// ================================================================================
// Automatically generated by   S5/S7 Converter,  Version K2.1.9.0-REL   12-04-2006 21:34
// ================================================================================
//
//                       Notes:
//                       ------
//
// BLOCKS:       The following block types exist in S7:
//OB: as in STEP 5;
//FB: function block (for example, closed-loop controller), is called using different instance data blocks;
//FC: function, similar to STEP 5 FBs.
//The block types PB, FX, DX and SB no longer exist.
//
//OBS:   OBs cannot be called from the user program in S7.
//        Special function OBs can be replaced by new instructions or by SFCs
//             in the same way as special instructions such as G DB.
//
// ADDRESSING: In S7, all memory areas (I, Q, M, D, etc.) can be addressed
//             as bytes. This means L DW 2 in S5 becomes L DBW 4 in S7.
//
// NO. OF ACCUS: All S7 CPUs have either 2 or 4 accumulators just as the S5 CPUs.
//               If an S5 program from an S5 CPU with 2 accumulators (S5-115U) is converted for an S7 CPU
//               with 4 accumulators, an ENT instruction must be added in front
//               of every math operation (+,-,*,/) in case the contents of accumulator 2
//               are to be used again afterwards.
//
// ACCU WIDTH: The accumulators of all S7 CPUs are 32 bits wide.
//             With fixed-point math operations in S7
//              - the high word in accumulator 1 remains unchanged following overflow/underflow
//                (S5-135U: sign);
//              - no implicit conversion to 32-bit format is performed (S5-155U).
//
// OS BIT:     With the following operations in S7, the OS bit
//             (stored overflow) remains unchanged (in S5 it was reset):
//             T,  >F, <F, ><F, !=F, >=F, <=F,  >D, <D, ><D, !=D, >=D, <=D,
//             >G, <G, ><G, !=G, >=G, <=G,
//             SLW, SRW, SLD, SSW, SSD, RLD, RRD
//
// OV BIT:      The following conversion operations leave the accumulator 1 unchanged
//              following an overflow (in S5: value of fixed-point number).
//              An overflow is displayed in the OS and OV bit (S5: only OS).
//              DUF, DUD, GFD
//
// LIR, TIR:    In S7 there are no instructions for absolute addressing. They are
//              partly replaced by new instructions (for example, access to data words greater than 255),
//              and partly by system functions (SFCs). The same applies to
//              data block start, data block length, and base register.
//
// DATA AREAS RS, RT, RI, RJ, Q:
//              When these data areas are used, the conversion requires manual assistance.
//              Possible solutions:
//                 - use the extended bit memory area
//                 - define longer data blocks
//                 - use S7 system functions (SFCs)
//
// STOP INSTRUCTIONS: In S7 there is only one stop instruction which can be executed by means of an
//               SFC call. It corresponds to the STS operation in S5.
//
// Refer to the manual or the on-line help for further information.


ORGANIZATION_BLOCK OB 1
VAR_TEMP
  OB1_EV_CLASS : BYTE ; //Bits 0-3 = 1 (Coming event), Bits 4-7 = 1 (Event class 1)
  OB1_SCAN_1 : BYTE ;   //1 (Cold restart scan 1 of OB 1), 3 (Scan 2-n of OB 1)
  OB1_PRIORITY : BYTE ; //1 (Priority of 1 is lowest)
  OB1_OB_NUMBR : BYTE ; //1 (Organization block 1, OB1)
  OB1_RESERVED_1 : BYTE ;   //Reserved for system
  OB1_RESERVED_2 : BYTE ;   //Reserved for system
  OB1_PREV_CYCLE : INT ;    //Cycle time of previous OB1 scan (milliseconds)
  OB1_MIN_CYCLE : INT ; //Minimum cycle time of OB1 (milliseconds)
  OB1_MAX_CYCLE : INT ; //Maximum cycle time of OB1 (milliseconds)
  OB1_DATE_TIME : DATE_AND_TIME ;   //Date and time OB1 started
  END_VAR
  BEGIN
  NETWORK
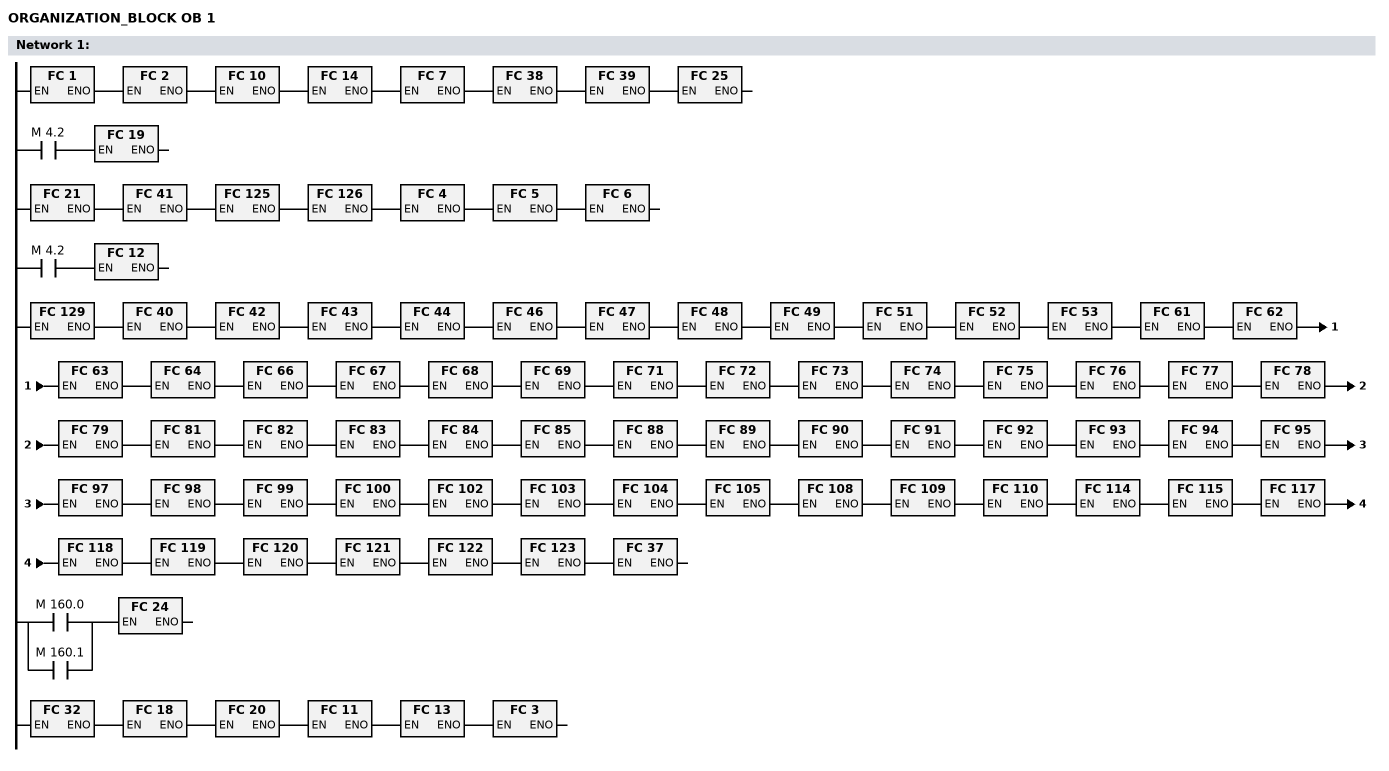
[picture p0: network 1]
       CALL FC 1;
       //;
       CALL FC 2;
       //;
       CALL FC 10;
       //;
       CALL FC 14;
       //;
       CALL FC 7;
       //;
       CALL FC 38;
       CALL FC 39;
       //;
       CALL FC 25;
       //;
       A   M 4.2;
       JCN   X000;
     CALL FC 19;
  X000: NOP 0;
       //;
       CALL FC 21;
       //;
       CALL FC 41;
       CALL FC 125;
       CALL FC 126;
       //;
       CALL FC 4;
       //;
       CALL FC 5;
       //;
       CALL FC 6;
       //;
       A   M 4.2;
       JCN   X001;
     CALL FC 12;
  X001: NOP 0;
       //;
       //;
       //;
       CALL FC 129;
       //;
       CALL FC 40;
       //;
       CALL FC 42;
       CALL FC 43;
       CALL FC 44;
       CALL FC 46;
       CALL FC 47;
       CALL FC 48;
       CALL FC 49;
       //;
       CALL FC 51;
       CALL FC 52;
       CALL FC 53;
       //;
       //;
       //;
       CALL FC 61;
       CALL FC 62;
       CALL FC 63;
       CALL FC 64;
       //;
       CALL FC 66;
       CALL FC 67;
       CALL FC 68;
       CALL FC 69;
       CALL FC 71;
       CALL FC 72;
       CALL FC 73;
       CALL FC 74;
       CALL FC 75;
       CALL FC 76;
       CALL FC 77;
       CALL FC 78;
       CALL FC 79;
       //;
       CALL FC 81;
       CALL FC 82;
       CALL FC 83;
       CALL FC 84;
       CALL FC 85;
       //;
       //;
       //;
       CALL FC 88;
       CALL FC 89;
       CALL FC 90;
       CALL FC 91;
       CALL FC 92;
       CALL FC 93;
       CALL FC 94;
       CALL FC 95;
       CALL FC 97;
       CALL FC 98;
       CALL FC 99;
       CALL FC 100;
       //;
       CALL FC 102;
       CALL FC 103;
       CALL FC 104;
       CALL FC 105;
       //;
       //;
       CALL FC 108;
       CALL FC 109;
       CALL FC 110;
       //;
       //;
       CALL FC 114;
       CALL FC 115;
       //;
       CALL FC 117;
       CALL FC 118;
       CALL FC 119;
       //;
       CALL FC 120;
       CALL FC 121;
       CALL FC 122;
       CALL FC 123;
       CALL FC 37;
       //;
       O   M 160.0;
       O   M 160.1;
       JCN   X002;
     CALL FC 24;
  X002: NOP 0;
       //;
       CALL FC 32;
       //;
       CALL FC 18;
       //;
       CALL FC 20;
       //;
       CALL FC 11;
       //;
       CALL FC 13;
       //;
       CALL FC 3;
       //;
  NETWORK


END_ORGANIZATION_BLOCK

ORGANIZATION_BLOCK OB 35
    // *** Warning in Line    5743:  Please check setting for time base (S7 Config.).
VAR_TEMP
  OB35_EV_CLASS : BYTE ;    //Bits 0-3 = 1 (Coming event), Bits 4-7 = 1 (Event class 1)
  OB35_STRT_INF : BYTE ;    //16#36 (OB 35 has started)
  OB35_PRIORITY : BYTE ;    //11 (Priority of 1 is lowest)
  OB35_OB_NUMBR : BYTE ;    //35 (Organization block 35, OB35)
  OB35_RESERVED_1 : BYTE ;  //Reserved for system
  OB35_RESERVED_2 : BYTE ;  //Reserved for system
  OB35_PHASE_OFFSET : WORD ;    //Phase offset (msec)
  OB35_RESERVED_3 : INT ;   //Reserved for system
  OB35_EXC_FREQ : INT ; //Frequency of execution (msec)
  OB35_DATE_TIME : DATE_AND_TIME ;  //Date and time OB35 started
  END_VAR
  BEGIN
  NETWORK
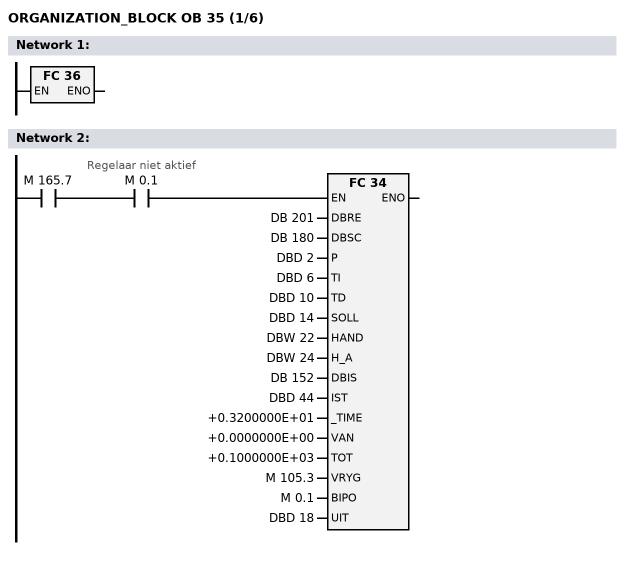
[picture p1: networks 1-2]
       CALL FC 36;
  NETWORK
       A   M 165.7;
       A   M 0.1;                // Regelaar niet aktief
       JCN   X000;

//  NAME: REGELAAR
//  VAR_INPUT
//    DBRE      :block_db;  // DBRE
//    DBSC      :block_db;  // DBSC
//    P         :dword;     // P
//    TI        :dword;     // TI
//    TD        :dword;     // TD
//    SOLL      :dword;     // SOLL
//    HAND      :word;      // HAND
//    H_A       :word;      // H/A
//    DBIS      :block_db;  // DBIS
//    IST       :dword;     // IST
//    _TIME     :real;      // TIME
//    VAN       :real;      // VAN
//    TOT       :real;      // TOT
//    VRYG      :bool;      // VRYG
//    BIPO      :bool;      // BIPO
//  END_VAR
//  VAR_OUTPUT
//    UIT       :dword;     // UIT
//  END_VAR



     CALL FC 34
        ( DBRE   :=  DB 201
        , DBSC   :=  DB 180
        , P      :=  DBD 2
        , TI     :=  DBD 6
        , TD     :=  DBD 10
        , SOLL   :=  DBD 14
        , HAND   :=  DBW 22
        , H_A    :=  DBW 24
        , DBIS   :=  DB 152
        , IST    :=  DBD 44
        , _TIME  :=  +0.3200000E+01
        , VAN    :=  +0.0000000E+00
        , TOT    :=  +0.1000000E+03
        , VRYG   :=  M 105.3
        , BIPO   :=  M 0.1
        , UIT    :=  DBD 18
        );
  X000: NOP 0;
  NETWORK
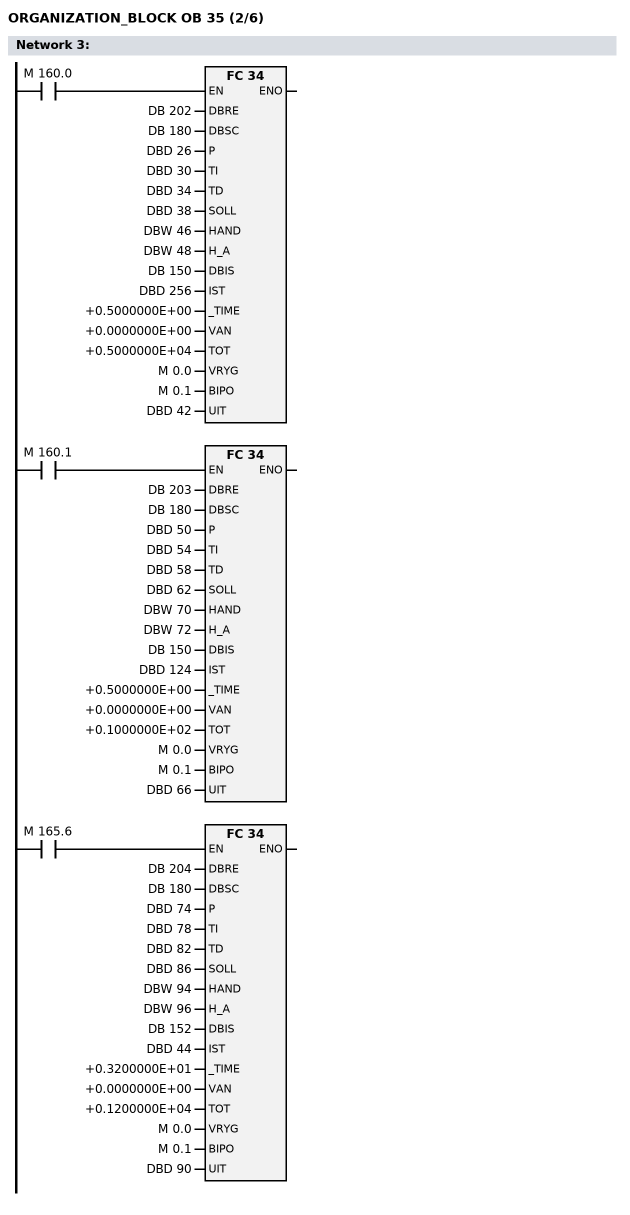
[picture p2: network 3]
       A   M 160.0;
       JCN   X001;
     CALL FC 34
        ( DBRE   :=  DB 202
        , DBSC   :=  DB 180
        , P      :=  DBD 26
        , TI     :=  DBD 30
        , TD     :=  DBD 34
        , SOLL   :=  DBD 38
        , HAND   :=  DBW 46
        , H_A    :=  DBW 48
        , DBIS   :=  DB 150
        , IST    :=  DBD 256
        , _TIME  :=  +0.5000000E+00
        , VAN    :=  +0.0000000E+00
        , TOT    :=  +0.5000000E+04
        , VRYG   :=  M 0.0
        , BIPO   :=  M 0.1
        , UIT    :=  DBD 42
        );
  X001: NOP 0;
       //;
       A   M 160.1;
       JCN   X002;
     CALL FC 34
        ( DBRE   :=  DB 203
        , DBSC   :=  DB 180
        , P      :=  DBD 50
        , TI     :=  DBD 54
        , TD     :=  DBD 58
        , SOLL   :=  DBD 62
        , HAND   :=  DBW 70
        , H_A    :=  DBW 72
        , DBIS   :=  DB 150
        , IST    :=  DBD 124
        , _TIME  :=  +0.5000000E+00
        , VAN    :=  +0.0000000E+00
        , TOT    :=  +0.1000000E+02
        , VRYG   :=  M 0.0
        , BIPO   :=  M 0.1
        , UIT    :=  DBD 66
        );
  X002: NOP 0;
       //;
       A   M 165.6;
       JCN   X003;
     CALL FC 34
        ( DBRE   :=  DB 204
        , DBSC   :=  DB 180
        , P      :=  DBD 74
        , TI     :=  DBD 78
        , TD     :=  DBD 82
        , SOLL   :=  DBD 86
        , HAND   :=  DBW 94
        , H_A    :=  DBW 96
        , DBIS   :=  DB 152
        , IST    :=  DBD 44
        , _TIME  :=  +0.3200000E+01
        , VAN    :=  +0.0000000E+00
        , TOT    :=  +0.1200000E+04
        , VRYG   :=  M 0.0
        , BIPO   :=  M 0.1
        , UIT    :=  DBD 90
        );
  X003: NOP 0;
  NETWORK
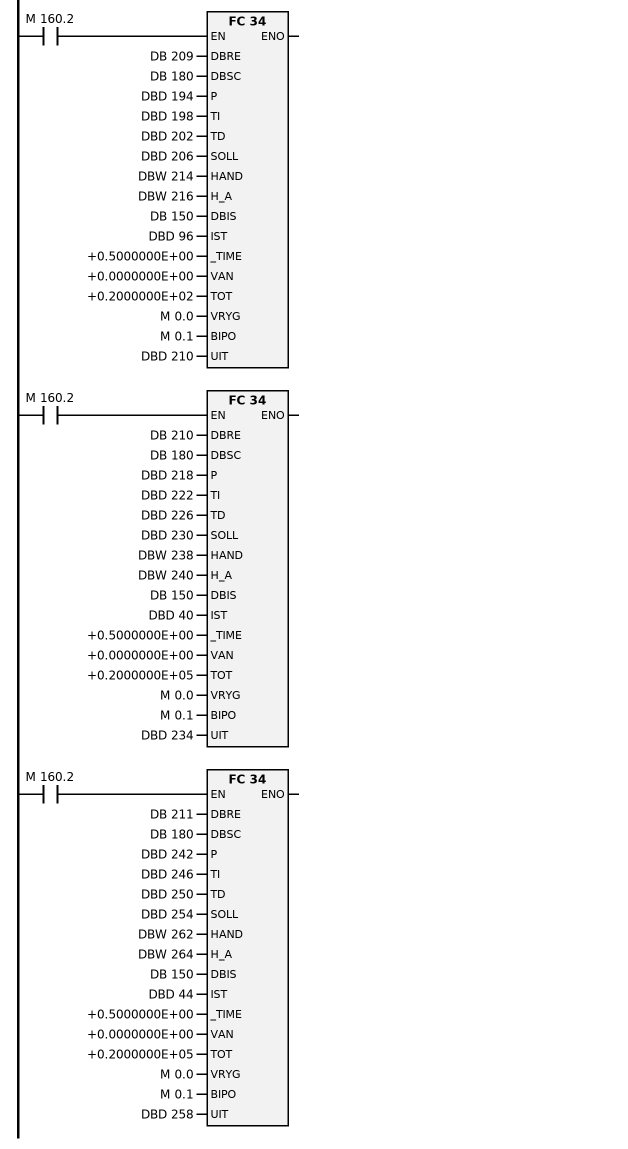
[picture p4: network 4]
       A   M 161.2;
       JCN   X004;
     CALL FC 34
        ( DBRE   :=  DB 206
        , DBSC   :=  DB 180
        , P      :=  DBD 122
        , TI     :=  DBD 126
        , TD     :=  DBD 130
        , SOLL   :=  DBD 134
        , HAND   :=  DBW 142
        , H_A    :=  DBW 144
        , DBIS   :=  DB 151
        , IST    :=  DBD 160
        , _TIME  :=  +0.8000000E+00
        , VAN    :=  +0.0000000E+00
        , TOT    :=  +0.1000000E+03
        , VRYG   :=  M 0.0
        , BIPO   :=  M 0.1
        , UIT    :=  DBD 138
        );
  X004: NOP 0;
       //;
       A   M 161.0;
       JCN   X005;
     CALL FC 34
        ( DBRE   :=  DB 207
        , DBSC   :=  DB 180
        , P      :=  DBD 146
        , TI     :=  DBD 150
        , TD     :=  DBD 154
        , SOLL   :=  DBD 158
        , HAND   :=  DBW 166
        , H_A    :=  DBW 168
        , DBIS   :=  DB 150
        , IST    :=  DBD 4
        , _TIME  :=  +0.8000001E+00
        , VAN    :=  +0.0000000E+00
        , TOT    :=  +0.1000000E+03
        , VRYG   :=  M 0.0
        , BIPO   :=  M 0.1
        , UIT    :=  DBD 162
        );
  X005: NOP 0;
       //;
       A   M 161.1;
       JCN   X006;
     CALL FC 34
        ( DBRE   :=  DB 208
        , DBSC   :=  DB 180
        , P      :=  DBD 170
        , TI     :=  DBD 174
        , TD     :=  DBD 178
        , SOLL   :=  DBD 182
        , HAND   :=  DBW 190
        , H_A    :=  DBW 192
        , DBIS   :=  DB 150
        , IST    :=  DBD 8
        , _TIME  :=  +0.8000001E+00
        , VAN    :=  +0.0000000E+00
        , TOT    :=  +0.1000000E+03
        , VRYG   :=  M 0.0
        , BIPO   :=  M 0.1
        , UIT    :=  DBD 186
        );
  X006: NOP 0;
       //;
       A   M 160.2;
       JCN   X007;
     CALL FC 34
        ( DBRE   :=  DB 209
        , DBSC   :=  DB 180
        , P      :=  DBD 194
        , TI     :=  DBD 198
        , TD     :=  DBD 202
        , SOLL   :=  DBD 206
        , HAND   :=  DBW 214
        , H_A    :=  DBW 216
        , DBIS   :=  DB 150
        , IST    :=  DBD 96
        , _TIME  :=  +0.5000000E+00
        , VAN    :=  +0.0000000E+00
        , TOT    :=  +0.2000000E+02
        , VRYG   :=  M 0.0
        , BIPO   :=  M 0.1
        , UIT    :=  DBD 210
        );
  X007: NOP 0;
       //;
       A   M 160.2;
       JCN   X008;
     CALL FC 34
        ( DBRE   :=  DB 210
        , DBSC   :=  DB 180
        , P      :=  DBD 218
        , TI     :=  DBD 222
        , TD     :=  DBD 226
        , SOLL   :=  DBD 230
        , HAND   :=  DBW 238
        , H_A    :=  DBW 240
        , DBIS   :=  DB 150
        , IST    :=  DBD 40
        , _TIME  :=  +0.5000000E+00
        , VAN    :=  +0.0000000E+00
        , TOT    :=  +0.2000000E+05
        , VRYG   :=  M 0.0
        , BIPO   :=  M 0.1
        , UIT    :=  DBD 234
        );
  X008: NOP 0;
       //;
       A   M 160.2;
       JCN   X009;
     CALL FC 34
        ( DBRE   :=  DB 211
        , DBSC   :=  DB 180
        , P      :=  DBD 242
        , TI     :=  DBD 246
        , TD     :=  DBD 250
        , SOLL   :=  DBD 254
        , HAND   :=  DBW 262
        , H_A    :=  DBW 264
        , DBIS   :=  DB 150
        , IST    :=  DBD 44
        , _TIME  :=  +0.5000000E+00
        , VAN    :=  +0.0000000E+00
        , TOT    :=  +0.2000000E+05
        , VRYG   :=  M 0.0
        , BIPO   :=  M 0.1
        , UIT    :=  DBD 258
        );
  X009: NOP 0;
  NETWORK
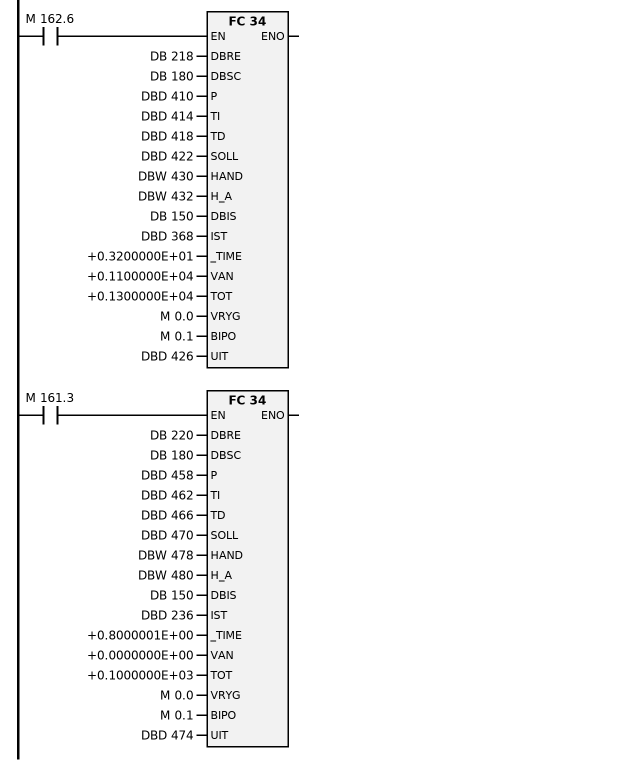
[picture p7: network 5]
       A   M 160.3;
       JCN   X010;
     CALL FC 34
        ( DBRE   :=  DB 212
        , DBSC   :=  DB 180
        , P      :=  DBD 266
        , TI     :=  DBD 270
        , TD     :=  DBD 274
        , SOLL   :=  DBD 278
        , HAND   :=  DBW 286
        , H_A    :=  DBW 288
        , DBIS   :=  DB 150
        , IST    :=  DBD 240
        , _TIME  :=  +0.5000000E+00
        , VAN    :=  +0.0000000E+00
        , TOT    :=  +0.1000000E+02
        , VRYG   :=  M 0.0
        , BIPO   :=  M 0.1
        , UIT    :=  DBD 282
        );
  X010: NOP 0;
       //;
       A   M 160.0;
       JCN   X011;
     CALL FC 34
        ( DBRE   :=  DB 213
        , DBSC   :=  DB 180
        , P      :=  DBD 290
        , TI     :=  DBD 294
        , TD     :=  DBD 298
        , SOLL   :=  DBD 302
        , HAND   :=  DBW 310
        , H_A    :=  DBW 312
        , DBIS   :=  DB 150
        , IST    :=  DBD 344
        , _TIME  :=  +0.5000000E+00
        , VAN    :=  +0.5500000E+01
        , TOT    :=  +0.8500000E+01
        , VRYG   :=  M 0.0
        , BIPO   :=  M 0.1
        , UIT    :=  DBD 306
        );
  X011: NOP 0;
       //;
       A   M 160.1;
       JCN   X012;
     CALL FC 34
        ( DBRE   :=  DB 214
        , DBSC   :=  DB 180
        , P      :=  DBD 314
        , TI     :=  DBD 318
        , TD     :=  DBD 322
        , SOLL   :=  DBD 326
        , HAND   :=  DBW 334
        , H_A    :=  DBW 336
        , DBIS   :=  DB 150
        , IST    :=  DBD 348
        , _TIME  :=  +0.5000000E+00
        , VAN    :=  +0.5500000E+01
        , TOT    :=  +0.8500000E+01
        , VRYG   :=  M 0.0
        , BIPO   :=  M 0.1
        , UIT    :=  DBD 330
        );
  X012: NOP 0;
       //;
       A   M 160.4;
       JCN   X013;
     CALL FC 34
        ( DBRE   :=  DB 215
        , DBSC   :=  DB 180
        , P      :=  DBD 338
        , TI     :=  DBD 342
        , TD     :=  DBD 346
        , SOLL   :=  DBD 350
        , HAND   :=  DBW 358
        , H_A    :=  DBW 360
        , DBIS   :=  DB 150
        , IST    :=  DBD 352
        , _TIME  :=  +0.5000000E+00
        , VAN    :=  +0.5500000E+01
        , TOT    :=  +0.8500000E+01
        , VRYG   :=  M 0.0
        , BIPO   :=  M 0.1
        , UIT    :=  DBD 354
        );
  X013: NOP 0;
       //;
       A   M 163.6;
       JCN   X014;
     CALL FC 34
        ( DBRE   :=  DB 216
        , DBSC   :=  DB 180
        , P      :=  DBD 362
        , TI     :=  DBD 366
        , TD     :=  DBD 370
        , SOLL   :=  DBD 374
        , HAND   :=  DBW 382
        , H_A    :=  DBW 384
        , DBIS   :=  DB 150
        , IST    :=  DBD 284
        , _TIME  :=  +0.3200000E+01
        , VAN    :=  +0.2000000E+01
        , TOT    :=  +0.1200000E+02
        , VRYG   :=  M 0.0
        , BIPO   :=  M 0.1
        , UIT    :=  DBD 378
        );
  X014: NOP 0;
       //;
       A   M 163.7;
       JCN   X015;
     CALL FC 34
        ( DBRE   :=  DB 217
        , DBSC   :=  DB 180
        , P      :=  DBD 386
        , TI     :=  DBD 390
        , TD     :=  DBD 394
        , SOLL   :=  DBD 398
        , HAND   :=  DBW 406
        , H_A    :=  DBW 408
        , DBIS   :=  DB 150
        , IST    :=  DBD 288
        , _TIME  :=  +0.3200000E+01
        , VAN    :=  +0.2000000E+01
        , TOT    :=  +0.1200000E+02
        , VRYG   :=  M 0.0
        , BIPO   :=  M 0.1
        , UIT    :=  DBD 402
        );
  X015: NOP 0;
       //;
       A   M 162.6;
       JCN   X016;
     CALL FC 34
        ( DBRE   :=  DB 218
        , DBSC   :=  DB 180
        , P      :=  DBD 410
        , TI     :=  DBD 414
        , TD     :=  DBD 418
        , SOLL   :=  DBD 422
        , HAND   :=  DBW 430
        , H_A    :=  DBW 432
        , DBIS   :=  DB 150
        , IST    :=  DBD 368
        , _TIME  :=  +0.3200000E+01
        , VAN    :=  +0.1100000E+04
        , TOT    :=  +0.1300000E+04
        , VRYG   :=  M 0.0
        , BIPO   :=  M 0.1
        , UIT    :=  DBD 426
        );
  X016: NOP 0;
       //;
       A   M 161.3;
       JCN   X017;
     CALL FC 34
        ( DBRE   :=  DB 220
        , DBSC   :=  DB 180
        , P      :=  DBD 458
        , TI     :=  DBD 462
        , TD     :=  DBD 466
        , SOLL   :=  DBD 470
        , HAND   :=  DBW 478
        , H_A    :=  DBW 480
        , DBIS   :=  DB 150
        , IST    :=  DBD 236
        , _TIME  :=  +0.8000001E+00
        , VAN    :=  +0.0000000E+00
        , TOT    :=  +0.1000000E+03
        , VRYG   :=  M 0.0
        , BIPO   :=  M 0.1
        , UIT    :=  DBD 474
        );
  X017: NOP 0;
  NETWORK
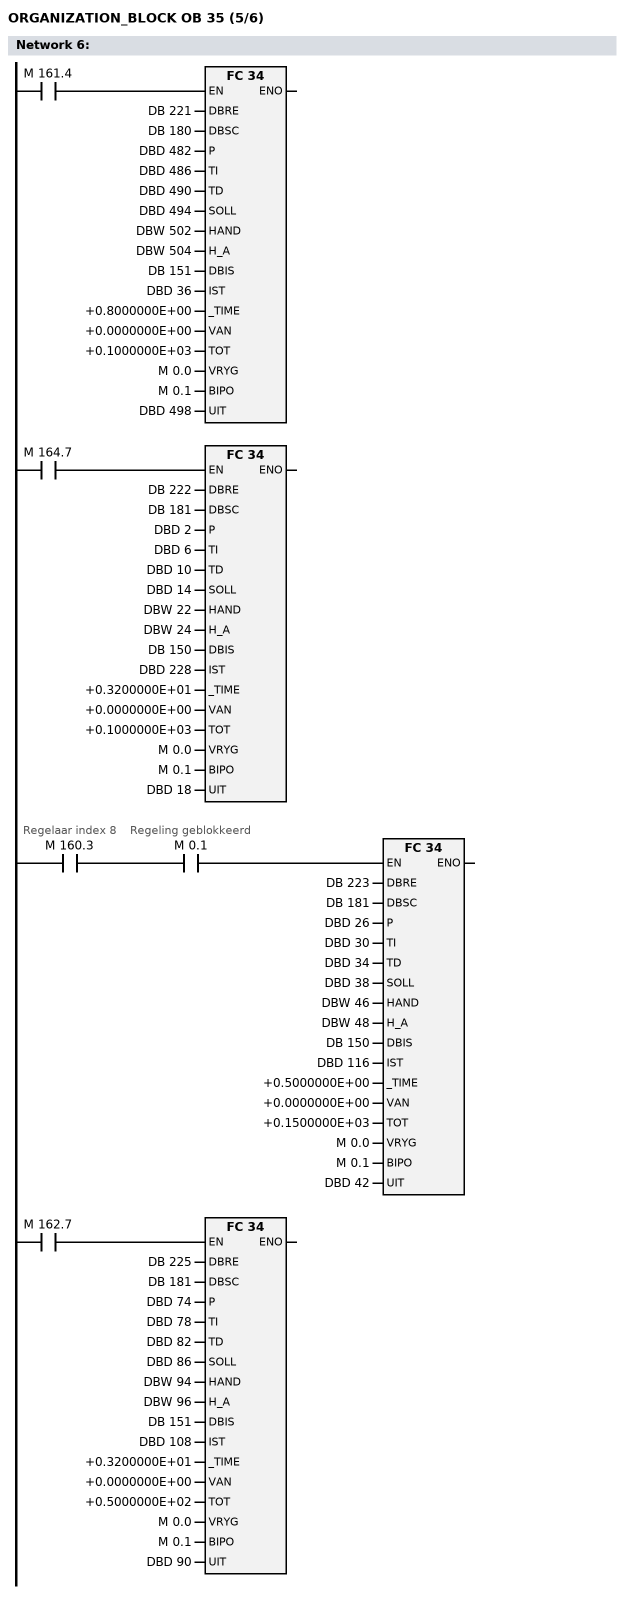
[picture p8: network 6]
       A   M 161.4;
       JCN   X018;
     CALL FC 34
        ( DBRE   :=  DB 221
        , DBSC   :=  DB 180
        , P      :=  DBD 482
        , TI     :=  DBD 486
        , TD     :=  DBD 490
        , SOLL   :=  DBD 494
        , HAND   :=  DBW 502
        , H_A    :=  DBW 504
        , DBIS   :=  DB 151
        , IST    :=  DBD 36
        , _TIME  :=  +0.8000000E+00
        , VAN    :=  +0.0000000E+00
        , TOT    :=  +0.1000000E+03
        , VRYG   :=  M 0.0
        , BIPO   :=  M 0.1
        , UIT    :=  DBD 498
        );
  X018: NOP 0;
       //;
       A   M 164.7;
       JCN   X019;
     CALL FC 34
        ( DBRE   :=  DB 222
        , DBSC   :=  DB 181
        , P      :=  DBD 2
        , TI     :=  DBD 6
        , TD     :=  DBD 10
        , SOLL   :=  DBD 14
        , HAND   :=  DBW 22
        , H_A    :=  DBW 24
        , DBIS   :=  DB 150
        , IST    :=  DBD 228
        , _TIME  :=  +0.3200000E+01
        , VAN    :=  +0.0000000E+00
        , TOT    :=  +0.1000000E+03
        , VRYG   :=  M 0.0
        , BIPO   :=  M 0.1
        , UIT    :=  DBD 18
        );
  X019: NOP 0;
       //;
       A   M 160.3;            // Regelaar index 8
       A   M 0.1;              // Regeling geblokkeerd
       JCN   X020;
     CALL FC 34                  // dPIC-160
        ( DBRE   :=  DB 223
        , DBSC   :=  DB 181
        , P      :=  DBD 26
        , TI     :=  DBD 30
        , TD     :=  DBD 34
        , SOLL   :=  DBD 38
        , HAND   :=  DBW 46
        , H_A    :=  DBW 48
        , DBIS   :=  DB 150
        , IST    :=  DBD 116
        , _TIME  :=  +0.5000000E+00
        , VAN    :=  +0.0000000E+00
        , TOT    :=  +0.1500000E+03
        , VRYG   :=  M 0.0
        , BIPO   :=  M 0.1
        , UIT    :=  DBD 42
        );
  X020: NOP 0;
       //;
       A   M 162.7;
       JCN   X021;
     CALL FC 34
        ( DBRE   :=  DB 225
        , DBSC   :=  DB 181
        , P      :=  DBD 74
        , TI     :=  DBD 78
        , TD     :=  DBD 82
        , SOLL   :=  DBD 86
        , HAND   :=  DBW 94
        , H_A    :=  DBW 96
        , DBIS   :=  DB 151
        , IST    :=  DBD 108
        , _TIME  :=  +0.3200000E+01
        , VAN    :=  +0.0000000E+00
        , TOT    :=  +0.5000000E+02
        , VRYG   :=  M 0.0
        , BIPO   :=  M 0.1
        , UIT    :=  DBD 90
        );
  X021: NOP 0;
  NETWORK
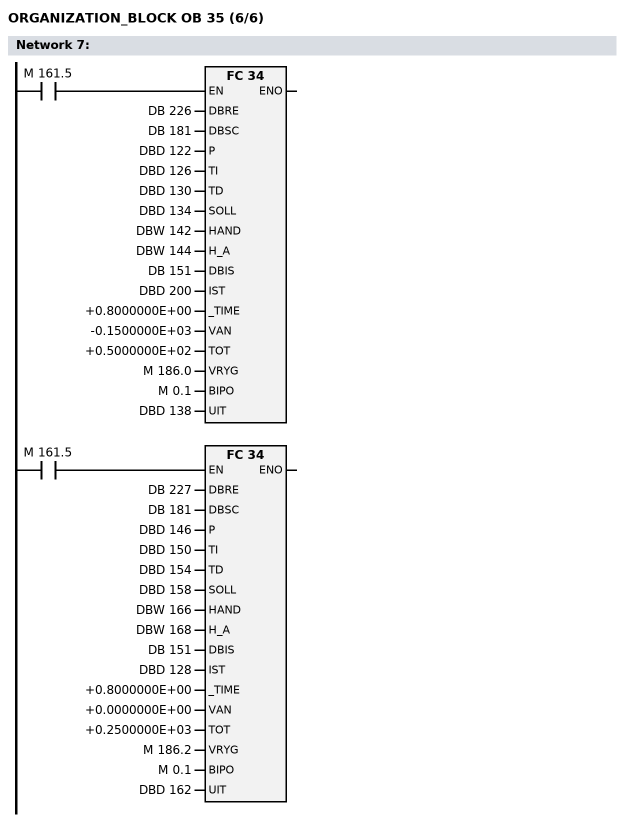
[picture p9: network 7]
       A   M 161.5;
       JCN   X022;
     CALL FC 34
        ( DBRE   :=  DB 226
        , DBSC   :=  DB 181
        , P      :=  DBD 122
        , TI     :=  DBD 126
        , TD     :=  DBD 130
        , SOLL   :=  DBD 134
        , HAND   :=  DBW 142
        , H_A    :=  DBW 144
        , DBIS   :=  DB 151
        , IST    :=  DBD 200
        , _TIME  :=  +0.8000000E+00
        , VAN    :=  -0.1500000E+03
        , TOT    :=  +0.5000000E+02
        , VRYG   :=  M 186.0
        , BIPO   :=  M 0.1
        , UIT    :=  DBD 138
        );
  X022: NOP 0;
       //;
       A   M 161.5;
       JCN   X023;
     CALL FC 34
        ( DBRE   :=  DB 227
        , DBSC   :=  DB 181
        , P      :=  DBD 146
        , TI     :=  DBD 150
        , TD     :=  DBD 154
        , SOLL   :=  DBD 158
        , HAND   :=  DBW 166
        , H_A    :=  DBW 168
        , DBIS   :=  DB 151
        , IST    :=  DBD 128
        , _TIME  :=  +0.8000000E+00
        , VAN    :=  +0.0000000E+00
        , TOT    :=  +0.2500000E+03
        , VRYG   :=  M 186.2
        , BIPO   :=  M 0.1
        , UIT    :=  DBD 162
        );
  X023: NOP 0;
  NETWORK


END_ORGANIZATION_BLOCK

ORGANIZATION_BLOCK OB 100
VAR_TEMP
  OB100_EV_CLASS : BYTE ;   //16#13, Event class 1, Entering event state, Event logged in diagnostic buffer
  OB100_STRTUP : BYTE ; //16#81/82/83/84 Method of startup
  OB100_PRIORITY : BYTE ;   //27 (Priority of 1 is lowest)
  OB100_OB_NUMBR : BYTE ;   //100 (Organization block 100, OB100)
  OB100_RESERVED_1 : BYTE ;  //Reserved for system
  OB100_RESERVED_2 : BYTE ; //Reserved for system
  OB100_STOP : WORD ;   //Event that caused CPU to stop (16#4xxx)
  OB100_STRT_INFO : DWORD ; //Information on how system started
  OB100_DATE_TIME : DATE_AND_TIME ; //Date and time OB100 started
  END_VAR
  BEGIN
  NETWORK
       CALL FC 9;
       //;
       CALL FC 33;
       //;
  NETWORK
       O   M 0.0;
       ON  M 0.0;
       S   M 5.0;
       S   M 5.1;
       S   M 5.2;


END_ORGANIZATION_BLOCK

ORGANIZATION_BLOCK OB 101
    // *** Warning in Line    6323:  If using an S5-115U, change to OB100.
VAR_TEMP
  OB101_EV_CLASS : BYTE ;   //16#13, Event class 1, Entering event state, Event logged in diagnostic buffer
  OB101_STRTUP : BYTE ; //16#81/82/83/84 Method of startup
  OB101_PRIORITY : BYTE ;   //27 (Priority of 1 is lowest)
  OB101_OB_NUMBR : BYTE ;   //101 (Organization block 101, OB101)
  OB101_RESERVED_1 : BYTE ; //Reserved for system
  OB101_RESERVED_2 : BYTE ; //Reserved for system
  OB101_STOP : WORD ;   //Event that caused CPU to stop (16#4xxx)
  OB101_STRT_INFO : DWORD ; //Information on how system started
  OB101_DATE_TIME : DATE_AND_TIME ; //Date and time OB101 started
  END_VAR
  BEGIN
  NETWORK
       CALL FC 9;
       //;
       CALL FC 33;
  NETWORK
       O   M 0.0;
       ON  M 0.0;
       S   M 5.0;
       S   M 5.1;
       S   M 5.2;


END_ORGANIZATION_BLOCK
//
// ORGANIZATION_BLOCK OB 22
//  // *** Error in Line    6350  (OB  22):   The program in the OB must be formulated differently (for example, using SFCs). ***
//VAR_TEMP
//  loc0: ARRAY [0..19] of BYTE;
//  END_VAR
//  BEGIN
//  NETWORK
//       CALL FC 9;
//       //;
//       CALL FC 33;
//  NETWORK
//       O   M 0.0;
//       ON  M 0.0;
//       S   M 5.0;
//       S   M 5.1;
//       S   M 5.2;
//
//
//END_ORGANIZATION_BLOCK

ORGANIZATION_BLOCK OB 81
    // *** Warning in Line    6371:  OB was interpreted as OB34 from S5-115U.
  AUTHOR: _24084
VAR_TEMP
  OB81_EV_CLASS : BYTE ;  //16#39, Event class 3, Entering event state, Internal fault event
  OB81_FLT_ID : BYTE ;  //16#XX, Fault identifcation code
  OB81_PRIORITY : BYTE ;    //26/28 (Priority of 1 is lowest)
  OB81_OB_NUMBR : BYTE ;    //81 (Organization block 81, OB81)
  OB81_RESERVED_1 : BYTE ;  //Reserved for system
  OB81_RESERVED_2 : BYTE ;  //Reserved for system
  OB81_MDL_ADDR : INT ; //Reserved for system
  OB81_RESERVED_3 : BYTE ;  //Reserved for system
  OB81_RESERVED_4 : BYTE ;  //Reserved for system
  OB81_RESERVED_5 : BYTE ;  //Reserved for system
  OB81_RESERVED_6 : BYTE ;  //Reserved for system
  OB81_DATE_TIME : DATE_AND_TIME ;  //Date and time OB81 started
  END_VAR
  BEGIN
  NETWORK


END_ORGANIZATION_BLOCK



